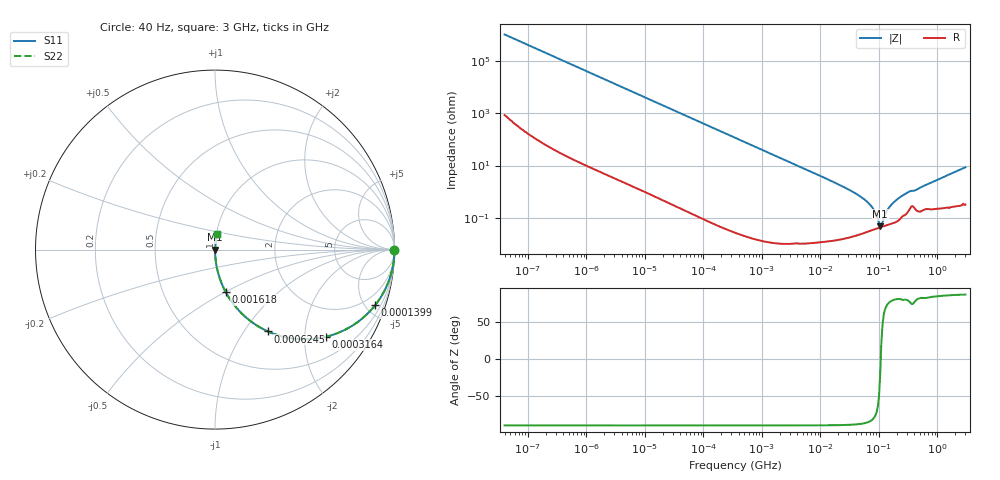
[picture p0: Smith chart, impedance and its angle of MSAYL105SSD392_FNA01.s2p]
! MSAYL105SSD392_FNA01  S-PARAMETER MODEL  ( General Type )
! Model Generated by TAIYO YUDEN Corporation (http://www.ty-top.com)
! Version 2.0
! TAIYO YUDEN Control No. 040624
! Copyright(c) 2004 TAIYO YUDEN CO.,LTD. All Rights Reserved.
! Product Description (link to TY-COMPAS)
! https://ds.yuden.co.jp/TYCOMPAS/or/detail?pn=MSAYL105SSD392KFNA01&u=M
! Products Name : Multilayer Ceramic Capacitors
! Characteristics :
!  Capacitance : 3900 pF , Rated Voltage : 10V
!  Case Size : 1.0 x 0.5 / 0.039 x 0.02 [mm/inch] , Thickness : 0.5 / 0.02 [mm/inch]
!  (Conditions: Temperature = 25 degC , DC Bias Current/Voltage = 0A / 0V)
! External Node Assignments :
!  1  o---| |---o  2
! GND o---------o GND
! Frequency Range : 40Hz  -  3GHz  [ 401 STEP ]
# MHz S RI R 50
! Freq[MHz].  S11 Real  S11 Imag  S21 Real  S21 Imag  S12 Real  S12 Imag  S22 Real  S22 Imag
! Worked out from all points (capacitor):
!   401 points, 40 Hz to 3 GHz, reference 50 ohm
!   read as one part in series: C = 3.94 nF near 44 Hz
!   lowest |Z| = 47.4 mohm at 104.8 MHz (marker M1)
!   series resonance near 107.3 MHz, so ESL is about 560 pH
!   S11 on the Smith chart (normalised r, x): 40 Hz: open; 139.9 kHz: 1.00, -5.77; 316.4 kHz: 1.00, -2.55; 624.5 kHz: 1.00, -1.29; 1.618 MHz: 1.00, -0.50; 3 GHz: 1.01, +0.17
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4e-05  1 -9.91e-05  9.3e-08 9.91e-05  9.3e-08 9.91e-05  1 -9.91e-05
0.000834  1 -0.00207  4.77e-06 0.00207  4.77e-06 0.00207  1 -0.00207
0.017386  0.9981 -0.043  0.00186 0.043  0.00186 0.043  0.9981 -0.043
0.054  0.9824 -0.1314  0.0176 0.1314  0.0176 0.1314  0.9824 -0.1314
0.139906  0.8927 -0.3094  0.1073 0.3094  0.1073 0.3094  0.8927 -0.3094
0.316385  0.6194 -0.4854  0.3806 0.4854  0.3806 0.4854  0.6194 -0.4854
0.362475  0.5536 -0.497  0.4464 0.497  0.4464 0.497  0.5536 -0.497
0.624497  0.2947 -0.4558  0.7053 0.4558  0.7053 0.4558  0.2947 -0.4558
0.982668  0.1444 -0.3514  0.8556 0.3514  0.8556 0.3514  0.1444 -0.3514
1.617971  0.0587 -0.2348  0.9413 0.2348  0.9413 0.2348  0.0587 -0.2348
7.222098  0.0032 -0.0555  0.9968 0.0555  0.9968 0.0555  0.0032 -0.0555
26.8909  0.00036 -0.014  0.9996 0.014  0.9996 0.014  0.00036 -0.014
53.07868  0.000288 -0.00565  0.9997 0.00565  0.9997 0.00565  0.000288 -0.00565
76.28187  0.000348 -0.00256  0.9997 0.00256  0.9997 0.00256  0.000348 -0.00256
104.7695  0.000438 -0.00018  0.9996 0.00018  0.9996 0.00018  0.000438 -0.00018
114.7124  0.000469 0.000479  0.9995 -0.000479  0.9995 -0.000479  0.000469 0.000479
131.4235  0.00052 0.00149  0.9995 -0.00149  0.9995 -0.00149  0.00052 0.00149
150.5692  0.000577 0.00253  0.9994 -0.00253  0.9994 -0.00253  0.000577 0.00253
206.7996  0.00078 0.00518  0.9992 -0.00518  0.9992 -0.00518  0.00078 0.00518
310.9844  0.00175 0.0093  0.9983 -0.0093  0.9983 -0.0093  0.00175 0.0093
427.1222  0.00218 0.0114  0.9978 -0.0114  0.9978 -0.0114  0.00218 0.0114
3000  0.0105 0.0848  0.9895 -0.0848  0.9895 -0.0848  0.0105 0.0848
